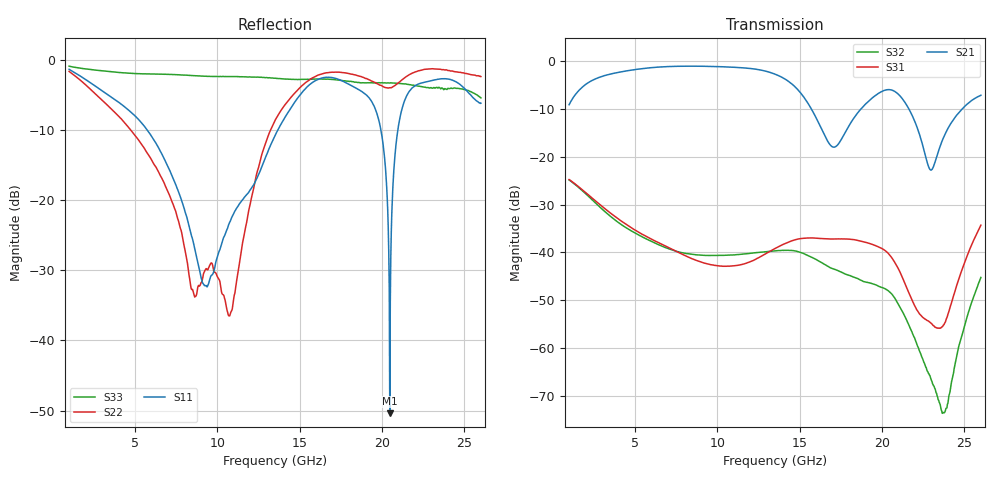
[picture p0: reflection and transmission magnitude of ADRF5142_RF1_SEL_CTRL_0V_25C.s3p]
! Device: ADRF5142
! Description: Silicon, SPDT Switch, Reflective
! Frequency: 8.00 GHz - 11.00 GHz
! Ports:
!  RFC = Port 1
!  RF1 = Port 2
!  RF2 = Port 3
! VDD = +3.3V
! VSS = -3.3V
! CTRL = 0V
! Temp = 25C
! Data:  Data was collected using an calibrated 4 port network analyzer.
!  The reference plane is the package pins of ADRF5142 switch.
! Notes: Analog Devices supplies this data as a sample of measured data
!  for this product.  Your particular data for this product may vary.
!  Data was taken at 25 degrees C.
!  Analog Devices reserves the right to change this data at anytime.
# HZ S DB R 50
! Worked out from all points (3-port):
!   801 points, 1 GHz to 26 GHz, reference 50 ohm
!   strongest paths, dB at 1 GHz, 7.25 GHz, 13.5 GHz, 19.75 GHz, 26 GHz:
!     S21: -9.1, -1.1, -2.7, -6.8, -7.1
!     S31: -24.8, -39.3, -39.2, -38.8, -34.3
!     S32: -24.8, -39.5, -39.7, -47.0, -45.2
!   lowest |S11| = -50.4 dB at 20.47 GHz (marker M1), VSWR 1.01, Z = 50.3 - j0.035 ohm
!   |S11| at or under -10 dB: 5.754 GHz to 13.66 GHz (7.909 GHz wide, 81.5 % of centre); 19.93 GHz to 20.95 GHz (1.022 GHz wide, 5 % of centre)
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1e9  -1.29 158.0  -9.09 37.7  -24.76 -39.1
     -9.09 37.7  -1.58 125.0  -24.84 -56.7
     -24.76 -39.1  -24.84 -56.7  -0.84 171.0
6.25e9  -11.75 89.1  -1.26 -94.1  -37.65 -124.6
        -1.26 -94.1  -15.15 -81.0  -38.09 133.1
        -37.65 -124.6  -38.09 133.1  -1.97 139.5
1.07187e10  -23.28 -151.6  -1.20 165.4  -42.87 -143.3
            -1.20 165.4  -36.49 117.9  -40.55 41.0
            -42.87 -143.3  -40.55 41.0  -2.31 111.5
1.35e10  -10.76 -113.4  -2.69 92.5  -39.18 -158.9
         -2.69 92.5  -8.60 70.3  -39.65 -26.5
         -39.18 -158.9  -39.65 -26.5  -2.55 95.0
1.65312e10  -2.45 170.0  -15.64 32.3  -37.13 139.3
            -15.64 32.3  -1.82 -32.4  -42.54 -126.6
            -37.13 139.3  -42.54 -126.6  -2.68 70.9
1.91562e10  -5.22 86.9  -8.42 60.5  -38.04 84.4
            -8.42 60.5  -2.73 -95.4  -46.30 151.1
            -38.04 84.4  -46.30 151.1  -3.21 50.4
2.04687e10  -50.40 -6.6  -5.94 11.1  -40.56 48.3
            -5.94 11.1  -3.91 -110.9  -48.29 92.8
            -40.56 48.3  -48.29 92.8  -3.23 39.2
2.125e10  -6.61 -174.7  -7.92 -25.3  -45.35 30.5
          -7.92 -25.3  -2.72 -113.8  -52.43 53.1
          -45.35 30.5  -52.43 53.1  -3.33 34.2
2.37187e10  -2.63 71.5  -16.06 22.3  -55.21 129.8
            -16.06 22.3  -1.32 -163.7  -73.49 -47.9
            -55.21 129.8  -73.49 -47.9  -4.11 8.4
2.6e10  -6.12 -22.4  -7.11 -27.8  -34.29 150.5
        -7.11 -27.8  -2.32 153.6  -45.23 158.6
        -34.29 150.5  -45.23 158.6  -5.36 -5.8
